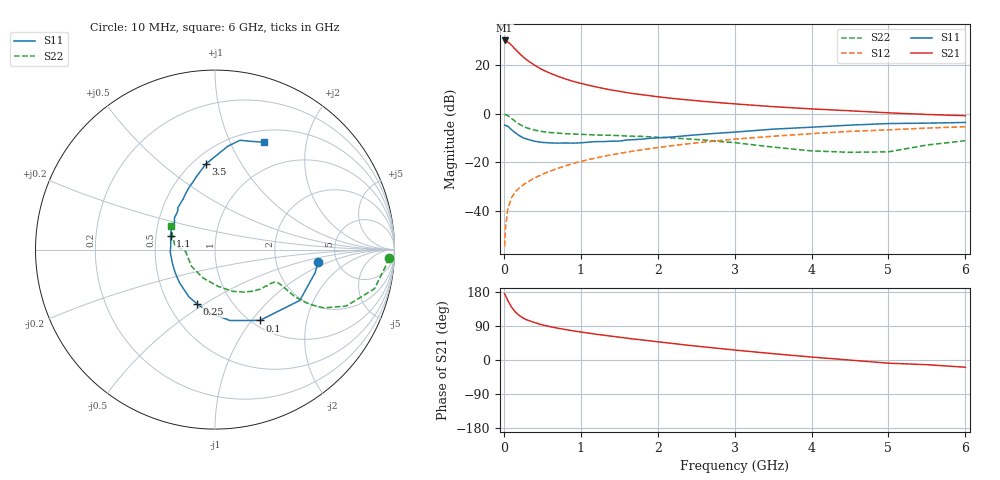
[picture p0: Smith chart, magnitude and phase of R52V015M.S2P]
! SIEMENS Small Signal Semiconductors
! BFR183
! Si NPN RF Bipolar Junction Transistor in SOT23
! VCE = 2 V  IC = 15 mA
! Common Emitter S-Parameters:  May  1996
# GHz  S  MA  R  50
!  f  S11  S21  S12  S22
! GHz  MAG  ANG  MAG  ANG  MAG  ANG  MAG  ANG
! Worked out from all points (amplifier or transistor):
!   36 points, 10 MHz to 6 GHz, reference 50 ohm
!   highest |S21| = 30.0 dB at 10 MHz (marker M1)
!   |S21| within 3 dB of that: start of sweep to 130.1 MHz
!   unconditionally stable (mu >= 1): 591.8 MHz to 2.416 GHz
!   at 250 MHz: K = 0.75, MSG = 26.3 dB, |S12| = -29.3 dB
!   at 1.4 GHz: K = 1.05, MAG = 11.9 dB, |S12| = -16.9 dB
!   at 6 GHz: K = 0.90, MSG = 2.3 dB, |S12| = -5.4 dB
!   S11 on the Smith chart (normalised r, x): 10 MHz: 3.59, -0.73; 100 MHz: 1.09, -1.10; 250 MHz: 0.69, -0.46; 1.1 GHz: 0.60, +0.10; 3.5 GHz: 0.58, +0.72; 6 GHz: 0.64, +1.35
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0.01  0.5788 -6.7  31.75 175.2  0.0019 92.7  0.9691 -2.8
0.02  0.5726 -13.0  31.33 170.4  0.0043 83.1  0.9546 -5.7
0.05  0.5509 -30.9  29.8 157.5  0.0107 79.0  0.9146 -13.8
0.1  0.4672 -57.6  25.35 139.6  0.0188 71.4  0.7969 -23.2
0.15  0.4041 -78.0  20.76 126.5  0.0249 66.6  0.6881 -28.2
0.2  0.3546 -94.4  17.35 117.6  0.0296 65.0  0.6085 -30.0
0.25  0.3186 -108.3  14.61 110.9  0.0343 65.3  0.5492 -30.5
0.3  0.3003 -119.1  12.6 105.8  0.0388 65.8  0.5089 -30.4
0.4  0.2707 -136.8  9.838 98.8  0.0478 67.1  0.4589 -29.3
0.5  0.2565 -149.9  7.977 92.7  0.0568 68.1  0.4275 -28.4
0.6  0.2502 -160.3  6.751 88.1  0.0657 68.6  0.409 -27.9
0.7  0.2475 -169.7  5.852 84.0  0.0751 69.1  0.3977 -27.8
0.8  0.2498 -176.6  5.145 80.4  0.0845 68.7  0.3874 -28.0
0.9  0.2474 175.2  4.599 77.0  0.0949 68.3  0.3808 -28.3
1.1  0.2592 163.0  3.826 71.0  0.1136 67.8  0.3703 -30.1
1.3  0.2667 153.4  3.268 65.4  0.1332 66.4  0.3606 -32.1
1.6  0.2874 141.8  2.694 57.6  0.162 63.8  0.3463 -36.3
2.2  0.3324 122.4  2.044 43.5  0.2206 57.9  0.3169 -46.9
3.5  0.4797 96.1  1.39 16.7  0.3431 41.7  0.2054 -85.3
4.5  0.58 83.0  1.143 -0.2  0.4321 28.9  0.1606 -144.8
5.5  0.6379 70.8  0.961 -12.4  0.5044 17.0  0.2267 173.1
6  0.6582 65.3  0.905 -19.1  0.5382 9.3  0.2782 152.2
